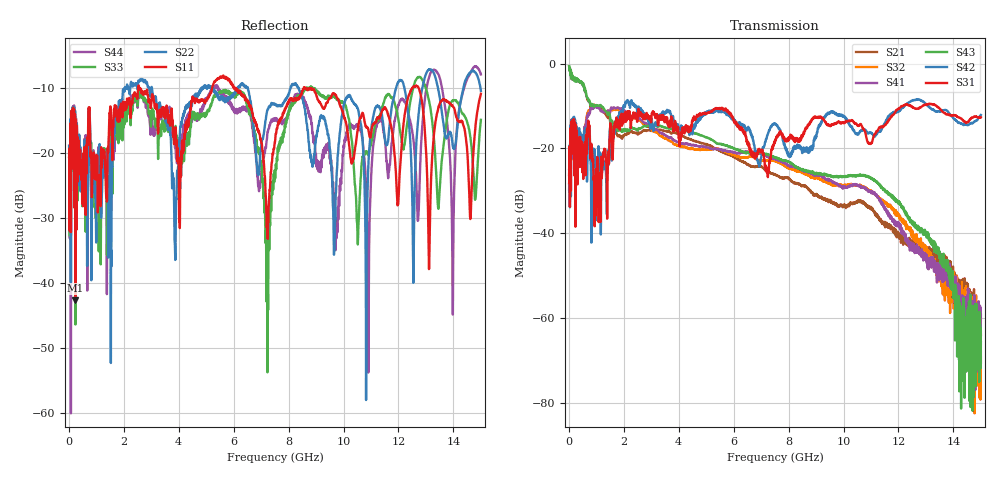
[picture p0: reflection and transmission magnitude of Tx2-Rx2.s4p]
! FILE: N:\QM 2007\Prüfprotokolle\Highspeed\Konfektionierte Ltg\L45593-D106\D30\8216\0002  kpl\IL  mit Chris Boards\Tx2-Rx2.s4p
# MHz S DB R 50.00
! FREQ  S11  S12  S13  S14
!  S21  S22  S23  S24
!  S31  S32  S33  S34
!  S41  S42  S43  S44
!  DB  ANG  DB  ANG  DB  ANG  DB  ANG
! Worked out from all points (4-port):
!   2999 points, 10 MHz to 15 GHz, reference 50 ohm
!   strongest paths, dB at 10 MHz, 3.755 GHz, 7.505 GHz, 11.26 GHz, 15 GHz:
!     S31: -26.3, -12.8, -18.4, -15.6, -12.7
!     S42: -24.9, -12.8, -14.1, -16.1, -12.1
!     S43: -0.6, -15.4, -22.1, -28.4, -65.8
!     S41: -29.8, -17.7, -22.6, -31.5, -59.3
!     S32: -28.3, -18.5, -23.0, -31.7, -70.6
!     S21: -0.6, -16.4, -26.1, -36.0, -64.1
!   lowest |S11| = -42.7 dB at 240 MHz (marker M1), VSWR 1.01, Z = 50.5 + j0.556 ohm
!   |S11| at or under -10 dB: start of sweep to 2.52 GHz; 2.562 GHz to 5.218 GHz (2.656 GHz wide, 68.3 % of centre); 8.779 GHz to 12.5 GHz (3.718 GHz wide, 35 % of centre)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
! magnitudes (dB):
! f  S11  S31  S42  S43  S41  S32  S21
! 10 MHz  -20.6  -26.3  -24.9  -0.6  -29.8  -28.3  -0.6
! 240 MHz  -42.7  -38.5  -28.1  -3.6  -16.4  -16.5  -3.6
! 7.23 GHz  -32.5  -25.3  -16.9  -21.4  -21.9  -23.0  -25.6
! 10.74 GHz  -14.6  -15.6  -15.4  -26.4  -29.4  -29.1  -32.7
! 13.35 GHz  -15.3  -9.9  -11.3  -43.4  -48.0  -47.5  -45.1
! 13.97 GHz  -12.8  -12.3  -12.7  -52.4  -50.9  -54.6  -49.1
! 15 GHz  -10.9  -12.7  -12.1  -65.8  -59.3  -70.6  -64.1
